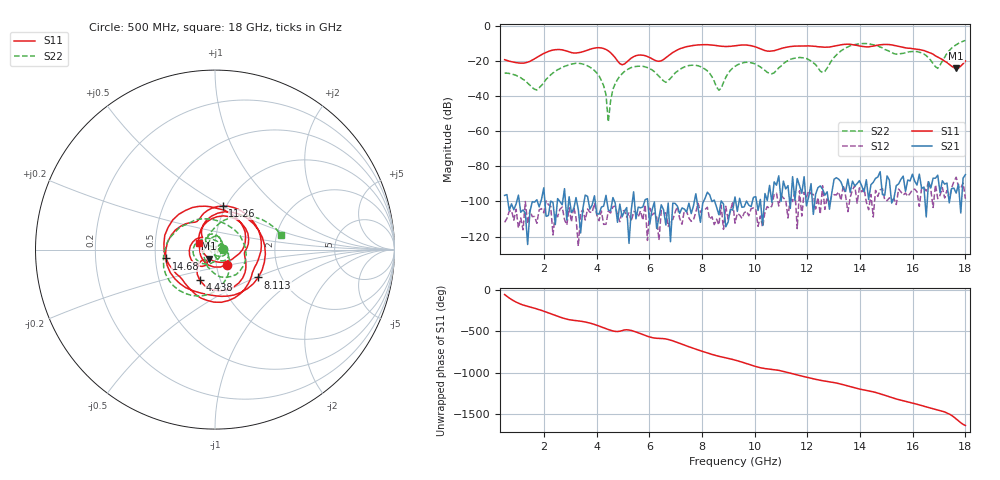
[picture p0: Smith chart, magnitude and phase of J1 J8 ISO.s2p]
!Agilent Technologies,N5230A,MY45001360,A.07.50.67
!Agilent N5230A: A.07.50.67
!Date: Tuesday, April 16, 2024 17:50:27
!Correction: S11(Full 2 Port(1,2))
!S21(Full 2 Port(1,2))
!S12(Full 2 Port(1,2))
!S22(Full 2 Port(1,2))
!S2P File: Measurements: S11, S21, S12, S22:
# Hz S  dB  R 50
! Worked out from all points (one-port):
!   201 points, 500 MHz to 18 GHz, reference 50 ohm
!   lowest |S11| = -24.4 dB at 17.65 GHz (marker M1), VSWR 1.13, Z = 46.5 - j4.69 ohm
!   |S11| at or under -10 dB: start of sweep to end of sweep
!   S11 on the Smith chart (normalised r, x): 500 MHz: 1.13, -0.19; 4.438 GHz: 0.80, -0.28; 8.113 GHz: 1.53, -0.52; 11.26 GHz: 0.96, +0.50; 14.68 GHz: 0.57, -0.06; 18 GHz: 0.83, +0.07
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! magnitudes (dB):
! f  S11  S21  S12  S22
! 500 MHz  -19.4  -96.5  -111.9  -27.1
! 1.725 GHz  -18.1  -99.0  -112.4  -36.6
! 3.475 GHz  -14.8  -103.7  -104.7  -21.9
! 4.263 GHz  -13.1  -102.6  -113.0  -34.2
! 4.438 GHz  -14.4  -104.8  -105.5  -54.7
! 4.612 GHz  -16.8  -97.8  -103.1  -36.3
! 5.05 GHz  -21.9  -105.7  -105.1  -26.2
! 6.362 GHz  -20.3  -109.2  -122.0  -28.9
! 8.113 GHz  -10.8  -98.2  -104.6  -24.8
! 8.637 GHz  -11.6  -107.5  -113.3  -36.8
! 9.25 GHz  -11.4  -97.4  -112.3  -23.2
! 10.65 GHz  -14.5  -100.4  -102.6  -27.4
! 11.26 GHz  -12.2  -91.0  -109.4  -19.9
! 12.22 GHz  -11.7  -107.3  -96.0  -21.2
! 12.57 GHz  -12.2  -92.9  -91.0  -26.7
! 13.45 GHz  -10.6  -94.3  -96.7  -12.7
! 14.68 GHz  -11.1  -86.1  -97.1  -11.6
! 15.11 GHz  -10.8  -87.8  -97.9  -14.7
! 16.34 GHz  -13.9  -92.5  -92.3  -15.6
! 16.95 GHz  -17.9  -85.1  -98.4  -24.3
! 17.65 GHz  -24.4  -95.2  -86.2  -10.9
! 18 GHz  -20.1  -84.7  -98.4  -8.5
